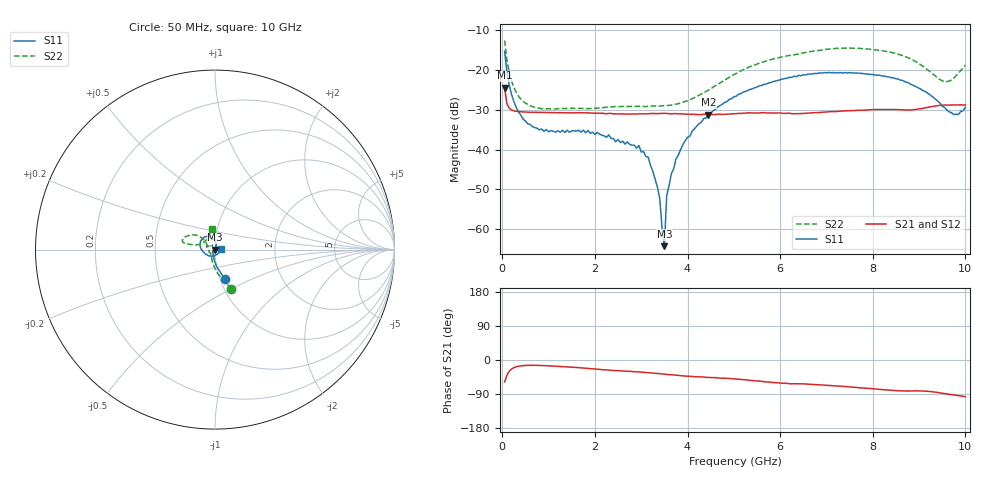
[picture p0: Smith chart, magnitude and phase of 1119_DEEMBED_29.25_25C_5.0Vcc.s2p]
!Hittite Microwave Corp.
!Digital Attenuator/PhaseShifter Rev 1.4.0
!Filename: C:\DATA\DATA\1119_DEEMBED_29.25_25C_5.0Vcc.s2p
!VNA ID: Agilent Technologies,N5224A,MY51441122,A.10.45.03
!Device type:
!2 Port Calibration.
!Temp(C): 25
!Lot Number:
!Serial Number:
!Operator:
!Misc:
!Attenuator:  29.250
# GHZ S DB R 50.0
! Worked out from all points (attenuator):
!   200 points, 50 MHz to 10 GHz, reference 50 ohm
!   highest |S21| = -24.46 dB at 50 MHz (marker M1); lowest = -31.2 dB at 4.45 GHz (marker M2)
!   lowest |S11| = -64.3 dB at 3.5 GHz (marker M3), VSWR 1.00, Z = 50.1 + j0.00809 ohm
!   |S11| at or under -10 dB: start of sweep to end of sweep
!   |S22| runs from -29.8 to -12.6 dB; largest |S21 - S12| = 0.00011
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0.05  -15.29 -71.6  -24.46 -58.3  -24.46 -58.3  -12.55 -67.5
0.1  -20.55 -84.8  -28.46 -40.2  -28.46 -40.1  -17.51 -84.0
0.2  -26.13 -97.3  -30.03 -23.9  -30.03 -23.8  -22.78 -100.6
0.55  -33.53 -122.1  -30.58 -14.1  -30.58 -14.2  -28.65 -126.4
0.9  -35.42 -133.7  -30.67 -14.7  -30.67 -14.8  -29.77 -135.9
1.75  -35.10 -139.3  -30.77 -21.3  -30.76 -21.4  -29.67 -140.9
2.95  -38.98 -112.0  -30.99 -31.4  -31.00 -31.5  -29.14 -160.2
3.15  -41.91 -102.4  -30.97 -33.1  -30.99 -33.2  -29.14 -166.2
3.4  -52.26 -103.0  -30.94 -36.0  -30.94 -36.0  -29.05 -173.8
3.45  -59.68 -46.2  -30.93 -36.7  -30.94 -36.7  -28.97 -175.7
3.5  -64.31 7.6  -30.88 -37.1  -30.88 -37.2  -28.94 -177.3
3.55  -51.60 62.0  -30.93 -38.3  -30.93 -38.3  -28.93 -179.2
3.75  -42.38 69.2  -30.96 -40.2  -30.98 -40.3  -28.58 173.0
4  -36.91 66.4  -31.12 -42.6  -31.13 -42.7  -27.76 161.8
4.45  -31.07 74.6  -31.23 -46.2  -31.24 -46.3  -25.06 146.1
5.05  -26.59 89.4  -30.96 -50.1  -30.97 -50.2  -20.83 138.6
6.7  -20.94 128.2  -30.74 -64.4  -30.75 -64.5  -15.26 153.8
8.35  -21.71 171.4  -29.94 -79.3  -29.94 -79.4  -15.44 168.1
9.15  -25.47 -144.2  -29.47 -82.3  -29.48 -82.3  -19.62 165.4
9.55  -29.41 -93.8  -28.81 -88.8  -28.82 -88.8  -22.88 138.1
9.75  -31.20 -50.7  -28.77 -92.2  -28.78 -92.2  -22.02 114.0
10  -29.38 4.4  -28.81 -96.7  -28.82 -96.7  -18.74 98.2
